// TwinCAT 3 PLC project PLCProject
// ProgramVersion: 3.1.4024.0
// libraries:
//   Tc2_Standard, * (Beckhoff Automation GmbH)
//   Tc2_System, * (Beckhoff Automation GmbH)
//   Tc3_Module, * (Beckhoff Automation GmbH)
// project tree:
//   / PlcTask.TcTTO
//   POUs/ MAIN.TcPOU
// real-time tasks:
//   TASK PlcTask: cycle T#10ms, priority 20, ADS port 350
// I/O:
//   DEVICE Device 3 (CX7000), AmsNetId 5.132.85.195.4.1
//     Term 1 (CX7028) [CX7028-0000-0118]
//       modules: Module 1 (DIO_2x), Module 3 (DIO_2x), Module 5 (DI_2x), Module 7 (DI_2x)
//   DEVICE Device 1 (EtherCAT), AmsNetId 5.132.85.195.2.1
//     Term 1 (EK1200) [EK1200-7000 EtherCAT Power supply (1,5A E-Bus)]
//       Term 2 (EL1859) [EL1859 8Ch. Dig. Input 24V, 3ms, 8Ch. Dig. Output 24V, 0.5A]
//       Term 3 (EL1859) [EL1859 8Ch. Dig. Input 24V, 3ms, 8Ch. Dig. Output 24V, 0.5A]
//       Term 4 (EL9011) [EL9011 End Terminal]

CONFIGURATION PLCProject
    RESOURCE PLC ON TwinCAT3
        TASK PlcTask(INTERVAL := T#10ms, PRIORITY := 20);
        PROGRAM MAIN WITH PlcTask : MAIN;
    END_RESOURCE
END_CONFIGURATION

// ---- POUs/MAIN.TcPOU
PROGRAM MAIN
VAR
END_VAR

// NETWORK 1

END_PROGRAM
